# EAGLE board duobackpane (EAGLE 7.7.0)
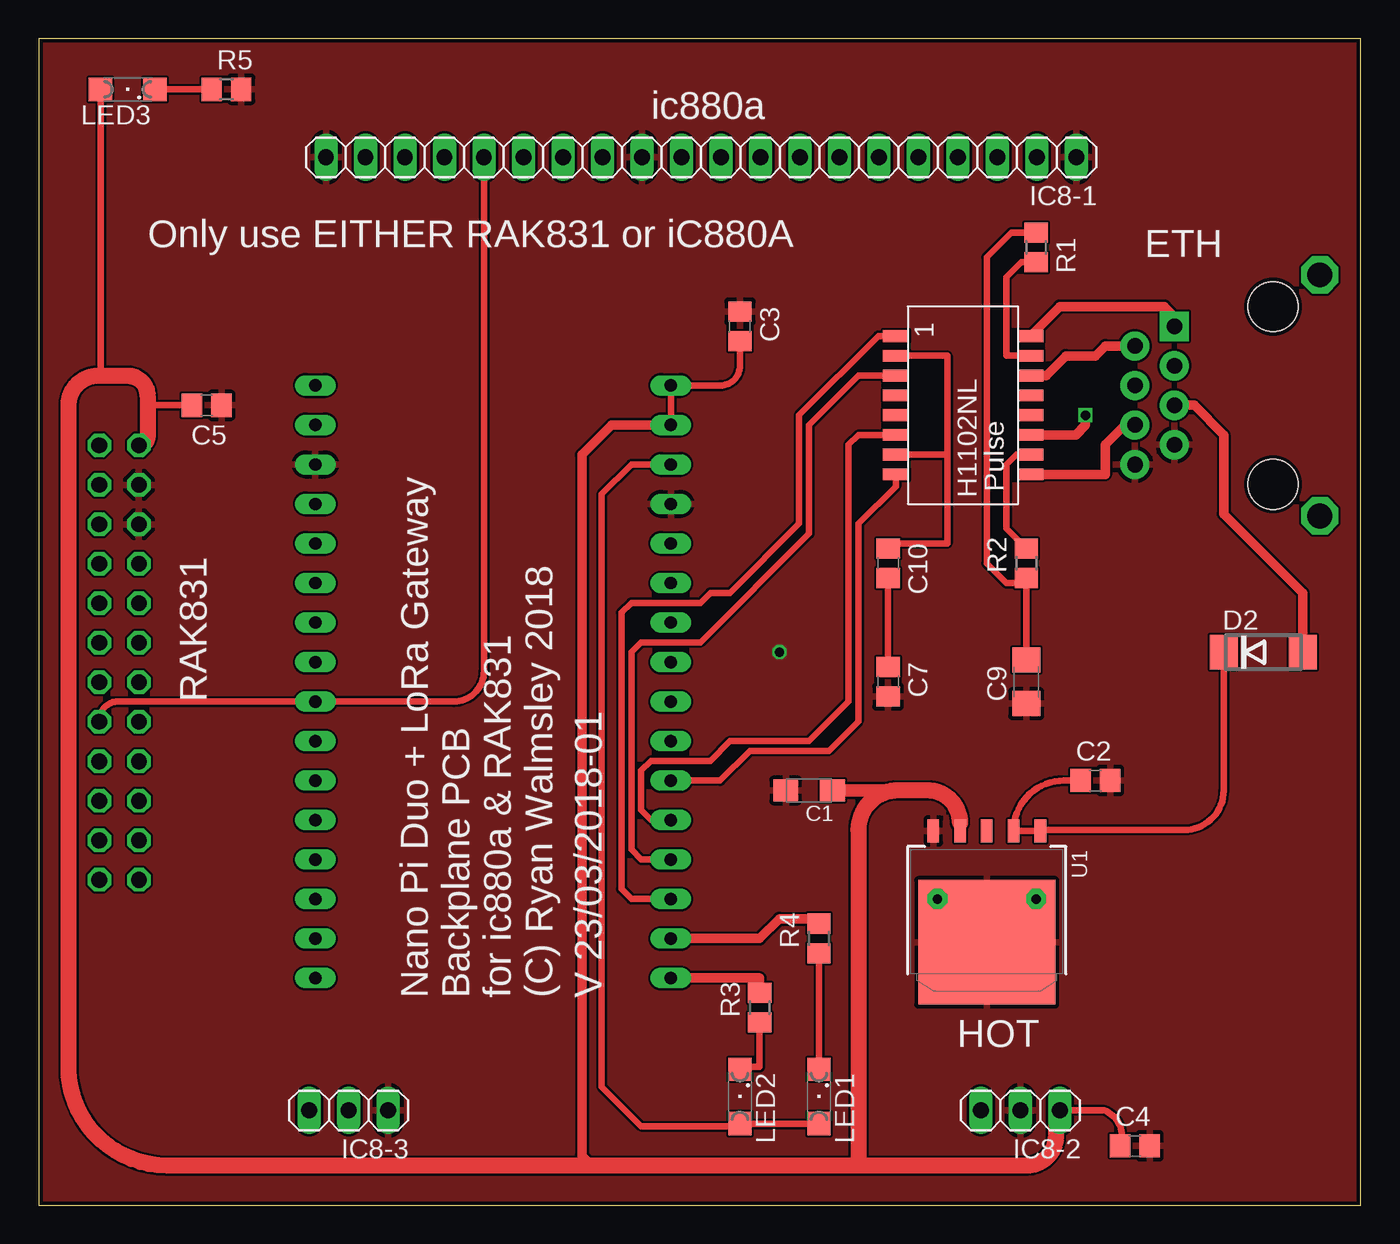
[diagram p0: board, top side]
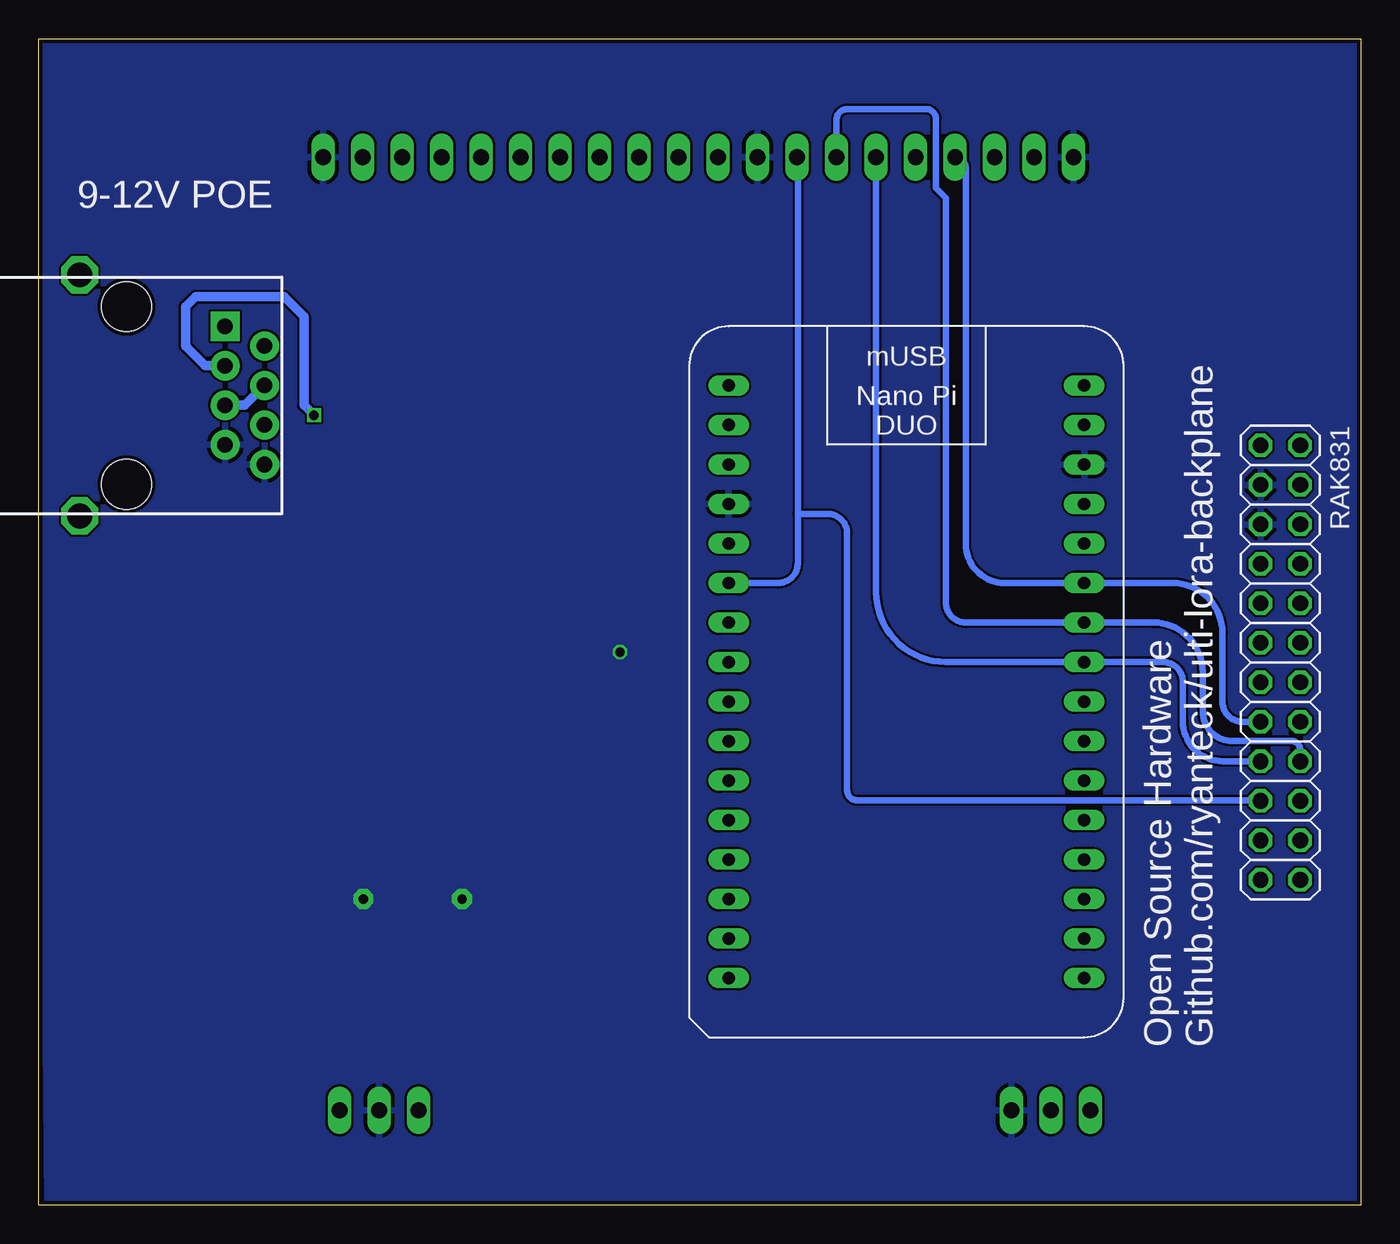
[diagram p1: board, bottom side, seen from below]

Size 85 x 75 mm. Coordinates in mm from the lower left corner, seen from the top.
Outline: 0,0 85,0 85,75 0,75 0,0
Copper layers (1*16): Top 0.035mm / dielectric 1.5mm / Bottom 0.035mm
Design rules "dirt_cheap_dirty_boards.v1.1": minimum track width 6mil, minimum drill 12mil, track to track 6mil, track to pad 6mil, pad to pad 6mil, via to via 6mil, smd to smd 0mil, copper to edge 10mil, drill to drill 10mil, minimum pad ring 10mil, minimum via ring 6mil, stop-mask expansion 2mil, vias tented up to drill 25mil, thermal gap 10mil

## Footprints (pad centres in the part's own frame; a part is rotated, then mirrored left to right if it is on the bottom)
SMC_A = smd 1.6 x 1.4: + -1.5,0; - 1.5,0
C0805 = smd 1.3 x 1.5: 1 -0.95,0; 2 0.95,0
C1206 = smd 1.6 x 1.8: 1 -1.4,0; 2 1.4,0
DO214AA = smd 1.8 x 2.2: A 2.55,0; C -2.55,0
1X20 = drill 1.016 long: 1 -24.13,0; 2 -21.59,0; 3 -19.05,0; 4 -16.51,0; 5 -13.97,0; 6 -11.43,0; 7 -8.89,0; 8 -6.35,0; 9 -3.81,0; 10 -1.27,0; 11 1.27,0; 12 3.81,0; 13 6.35,0; 14 8.89,0; 15 11.43,0; 16 13.97,0; 17 16.51,0; 18 19.05,0; 19 21.59,0; 20 24.13,0
1X03 = drill 1.016 long: 1 -2.54,0; 2 0,0; 3 2.54,0
RJ45-8 = drill 1 pad 1.88 square: 1 -4.445,6.35 | drill 1 pad 1.88: 2 -3.175,8.89; 3 -1.905,6.35; 4 -0.635,8.89; 5 0.635,6.35; 6 1.905,8.89; 7 3.175,6.35; 8 4.445,8.89 | drill 1.6 octagon: P$1 7.75,-3; P$2 -7.75,-3 | hole 3.2: -5.715,0; 5.715,0
SML1206 = smd 1.5 x 1.5: A 1.75,0; C -1.75,0
R0805 = smd 1.3 x 1.5: 1 -0.95,0; 2 0.95,0
2X12 = drill 1.016 octagon: 1 -13.97,-1.27; 2 -13.97,1.27; 3 -11.43,-1.27; 4 -11.43,1.27; 5 -8.89,-1.27; 6 -8.89,1.27; 7 -6.35,-1.27; 8 -6.35,1.27; 9 -3.81,-1.27; 10 -3.81,1.27; 11 -1.27,-1.27; 12 -1.27,1.27; 13 1.27,-1.27; 14 1.27,1.27; 15 3.81,-1.27; 16 3.81,1.27; 17 6.35,-1.27; 18 6.35,1.27; 19 8.89,-1.27; 20 8.89,1.27; 21 11.43,-1.27; 22 11.43,1.27; 23 13.97,-1.27; 24 13.97,1.27
HRP5 = smd 0.75 x 1.5: 1 -3.44,-1.2; 2 -1.72,-1.2; 3 0,-1.2; 4 1.72,-1.2; 5 3.44,-1.2 | smd 8.8 x 8: 6 0,5.96
DECADE-H1102NL = smd 0.76 x 1.67: 1 1.9,-0.77; 2 3.17,-0.77; 3 4.44,-0.77; 4 5.71,-0.77; 5 6.98,-0.77; 6 8.25,-0.77; 7 9.52,-0.77; 8 10.79,-0.77; 9 10.79,7.87; 10 9.52,7.87; 11 8.25,7.87; 12 6.98,7.87; 13 5.71,7.87; 14 4.44,7.87; 15 3.17,7.87; 16 1.9,7.87
NANOPIDUO = drill 0.8 long: 3V3 22.86,5.08; 5V@1 22.86,0; 5V@2 22.86,2.54; CLK 0,15.24; CS 0,12.7; CVB 0,27.94; DM2 22.86,20.32; DM3 22.86,15.24; DP2 22.86,22.86; DP3 22.86,17.78; DRX 0,0; DTX 0,2.54; GND 0,5.08; GND@2 22.86,7.62; IOG11 22.86,12.7; IRRX 22.86,10.16; LNK 22.86,35.56; LOL 0,30.48; LOR 0,33.02; MICN 0,38.1; MICP 0,35.56; MISO 0,17.78; MOSI 0,20.32; RD+ 22.86,27.94; RD- 22.86,25.4; RX1 0,22.86; SCL 0,7.62; SDA 0,10.16; SPD 22.86,38.1; TD+ 22.86,33.02; TD- 22.86,30.48; TX1 0,25.4

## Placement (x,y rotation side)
C1  [SMC_A]  49.53,26.67 180 top
C2  [C0805]  67.94,27.3 0 top
C3  [C0805]  45.09,56.52 270 top
C4  [C0805]  70.48,3.81 0 top
C5  [C0805]  10.79,51.44 180 top
C7  0.01uF  [C0805]  54.61,33.66 270 top
C9  1000pF 2kv  [C1206]  63.5,33.66 90 top
C10  0.01uF  [C0805]  54.61,41.27 270 top
D2  VS-10BQ060-M3/5BT  [DO214AA]  78.74,35.56 0 top
IC8-1  [1X20]  42.59,67.39 180 top
IC8-2  [1X03]  63.12,6.09 180 top
IC8-3  [1X03]  19.92,6.09 180 top
J1  RJ45-8PTH  [RJ45-8]  79.38,52.07 270 bottom
LED1  LNK  [SML1206]  50.16,6.99 270 top
LED2  SPD  [SML1206]  45.09,6.99 270 top
LED3  PWR  [SML1206]  5.71,71.75 180 top
R1  75R  [R0805]  64.14,61.59 270 top
R2  75R  [R0805]  63.5,41.27 90 top
R3  330R  [R0805]  46.35,12.7 90 top
R4  330R  [R0805]  50.16,17.14 90 top
R5  1K  [R0805]  12.06,71.75 0 top
RAK831  [2X12]  5.16,34.89 270 bottom
U1  BAXXDD0XX  [HRP5]  60.96,22.86 180 top
U$1  DECADE-H1102NL  [DECADE-H1102NL]  55.88,57.78 270 top
U$2  NANOPIDUO  [NANOPIDUO]  17.78,52.7 180 bottom

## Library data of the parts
C1-C5 C7 C9 C10 R1-R5 = resistor
D2 = diode
IC8-1-IC8-3 RAK831 = pinhead
J1 = decade
LED1-LED3 = led
U1 = rohm-semi
U$1 = DECADE-libraries20151104
U$2 = ryanteck

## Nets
+3V3: LED1.A LED2.A U$2.3V3
+5V: C1.+ C3.2 C4.1 C5.2 IC8-2.1 LED3.A RAK831.1 U1.4 U$2.5V@1 U$2.5V@2
GND: C1.- C2.2 C3.1 C4.2 C5.1 C7.2 C9.1 IC8-1.1 IC8-1.12 IC8-1.20 IC8-2.2 IC8-3.1 J1.7 J1.8 R5.2 RAK831.3 RAK831.5 U1.5 U1.6 U$2.GND U$2.GND@2
GPIO_RST: IC8-1.13 RAK831.19 U$2.IOG11
MISO: IC8-1.15 RAK831.17 U$2.MISO
MOSI: IC8-1.16 RAK831.16 U$2.MOSI
N$1: C2.1 D2.C U1.1 U1.2
N$2: R3.2 U$2.SPD
N$3: R4.2 U$2.LNK
N$4: LED2.C R3.1
N$5: R2.2 U$1.10
N$6: C9.2 R1.1 R2.1
N$7: LED1.C R4.1
N$8: C7.1 C10.2
N$9: LED3.C R5.1
N$13: C10.1 U$1.2 U$1.7
N$21: R1.2 U$1.15
NSS: IC8-1.17 RAK831.15 U$2.CS
RD+: U$1.6 U$2.RD+
RD-: U$1.8 U$2.RD-
RX+: J1.3 U$1.11
RX-: J1.6 U$1.9
SCLK: IC8-1.14 RAK831.18 U$2.CLK
TD+: U$1.1 U$2.TD+
TD-: U$1.3 U$2.TD-
TX+: J1.1 U$1.16
TX-: J1.2 U$1.14
VCC: D2.A J1.4 J1.5

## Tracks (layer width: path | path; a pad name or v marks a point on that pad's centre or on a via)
+3V3
  Top 0.406: U$2.3V3 38.1,47.62 36.2,45.72 36.2,7.62 38.73,5.08 44.93,5.08 LED2.A LED1.A
+5V
  Top 0.406: U1.4 59.24,24.58 | U$2.5V@2 U$2.5V@1 43.81,52.7 arc90 45.09,53.98 C3.2 | 6.99,52.07 arc90 7.62,51.44 C5.2 | C4.1 arc90 68.53,6.09 IC8-2.1 | LED3.A 3.96,53.49 3.81,53.34
  Top 0.61: U$2.5V@2 36.83,50.16 34.92,48.26 34.92,3.17 35.56,2.54
  Top 0.813: C1.+ 55.24,26.67
  Top 1.016: IC8-2.1 arc-90 65.41,6.34 65.41,4.45 arc-90 63.5,2.54 52.7,2.54 | 52.7,2.54 35.56,2.54 8.26,2.54 arc-90 1.91,8.89 1.91,51.44 arc-90 3.81,53.34 5.71,53.34 arc-90 6.99,52.07 6.99,49.41 arc-90 RAK831.1 | 59.24,24.58 arc90 57.15,26.67 55.24,26.67 arc90 52.7,24.13 52.7,2.54
GND  (via drill 0.6, 0.6 pad 1.27)
  other vias: 64.14,19.68 57.78,19.68 47.62,35.56
  pour Top: -3.81,-1.27 -3.81,5.08 -2.54,76.2 85.09,75.56 85.09,-0.64 -1.27,-1.27
  pour Bottom: -2.54,0.64 -5.08,-0.64 -1.27,74.93 85.09,75.56 85.09,71.75 84.45,0 -1.91,-0.64
GPIO_RST
  Bottom 0.406: IC8-1.13 arc90 36.2,67.34 36.2,44.45 | 36.2,44.45 36.2,41.27 arc90 37.47,40.01 U$2.IOG11 | RAK831.19 arc-90 6.46,26.04 32.38,26.04 arc90 33.02,26.67 33.02,43.18 arc-90 34.29,44.45 36.2,44.45
MISO
  Bottom 0.406: RAK831.17 8.86,28.54 arc90 11.43,31.11 11.43,33.66 arc-90 12.7,34.92 U$2.MISO 26.67,34.92 arc90 31.16,39.41 IC8-1.15
MOSI
  Top 0.406: RAK831.16 3.89,31.2 arc-90 5.08,32.38 U$2.MOSI 26.67,32.38 arc90 28.62,34.34 IC8-1.16
N$1
  Top 0.406: D2.C 76.19,26.66 arc-90 73.66,24.13 64.47,24.13 arc90 U1.1 U1.2 arc-90 65.92,27.3 C2.1
N$2
  Top 0.61: R3.2 46.35,14.61 U$2.SPD
N$3
  Top 0.61: U$2.LNK 46.35,17.14 47.62,18.41 49.84,18.41 R4.2
N$4
  Top 0.406: R3.1 46.35,8.89 45.09,8.89 LED2.C
N$5
  Top 0.406: U$1.10 62.87,48.27 62.23,47.62 62.23,43.49 R2.2
N$6
  Top 0.406: R1.1 62.55,62.55 60.96,60.96 60.96,41.27 62.23,40.01 63.18,40.01 R2.1 C9.2
N$7
  Top 0.406: R4.1 LED1.C
N$8
  Top 0.406: C7.1 C10.2
N$9
  Top 0.406: LED3.C R5.1
N$13
  Top 0.406: U$1.7 58.42,48.27 | 58.42,48.27 58.42,42.55 54.61,42.55 C10.1 | U$1.2 58.42,54.62 58.42,48.27
N$21
  Top 0.406: U$1.15 62.23,54.62 62.23,59.69 63.19,60.65 R1.2
NSS
  Bottom 0.406: RAK831.15 7.58,31.08 arc90 8.89,32.38 8.89,36.83 arc-90 12.06,40.01 U$2.CS 22.86,40.01 arc90 25.4,42.55 25.4,66.71 arc-90 IC8-1.17
RD+
  Top 0.406: U$2.RD+ 39.37,24.77 38.73,25.4 38.73,27.94 39.37,28.57 43.18,28.57 44.45,29.84 49.53,29.84 52.07,32.38 52.07,48.9 52.71,49.53 U$1.6
RD-
  Top 0.406: U$1.8 55.11,46.22 52.7,43.81 52.7,31.11 50.8,29.21 45.72,29.21 43.81,27.3 U$2.RD-
RX+  (via drill 0.6)
  Top 0.61: v67.31,50.8 67.31,50.16 66.67,49.53 U$1.11
  Bottom 0.61: J1.3 74.3,53.98 75.56,55.24 75.56,57.78 74.93,58.42 69.22,58.42 67.94,57.15 67.94,51.44 v67.31,50.8
RX-
  Top 0.61: J1.6 69.85,50.16 68.58,48.9 68.58,46.99 U$1.9
SCLK
  Bottom 0.406: RAK831.18 3.89,29.29 arc-90 4.45,29.84 8.26,29.84 arc90 10.16,31.75 10.16,34.29 arc-90 13.34,37.47 U$2.CLK 25.4,37.47 arc90 26.67,38.73 26.67,64.77 27.3,65.41 27.3,69.85 arc-90 27.94,70.48 33.02,70.48 arc-90 33.7,69.81 IC8-1.14
TD+
  Top 0.406: U$1.1 53.98,55.88 48.9,50.8 48.9,43.81 44.45,39.37 43.18,39.37 42.55,38.73 38.1,38.73 37.47,38.1 37.47,20.32 38.1,19.68 U$2.TD+
TD-
  Top 0.406: U$1.3 52.71,53.34 49.53,50.16 49.53,43.18 42.55,36.2 38.73,36.2 38.1,35.56 38.1,22.86 38.73,22.23 U$2.TD-
TX+
  Top 0.61: J1.1 73.03,57.15 72.39,57.78 65.65,57.78 U$1.16
TX-
  Top 0.61: U$1.14 64.78,53.34 66.04,54.61 67.94,54.61 68.58,55.24 J1.2
VCC
  Top 0.61: J1.5 74.3,51.44 76.2,49.53 76.2,44.45 81.28,39.37 D2.A
  Bottom 0.61: J1.4 71.75,51.44 J1.5

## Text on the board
tNames: ic880a | Only use EITHER RAK831 or iC880A | ETH | RAK831 | Nano Pi Duo + LoRa Gateway / Backplane PCB / for ic880a & RAK831 / (C) Ryan Walmsley 2018 | V 23/03/2018-01 | HOT
bNames: 9-12V POE | Open Source Hardware / Github.com/ryanteck/ulti-lora-backplane

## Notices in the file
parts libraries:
DECADE-libraries20151104: Licensing: Creative Commons ShareAlike 4.0 International - https://creativecommons.org/licenses/by-sa/4.0
rohm-semi: Copyright (C) 2010, Bob Starr
